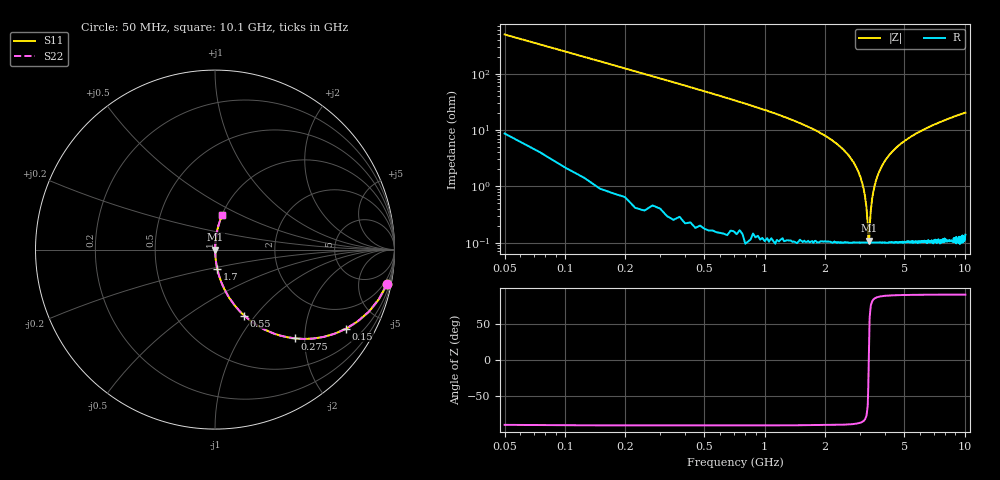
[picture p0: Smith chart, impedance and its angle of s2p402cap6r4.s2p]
! AVX Thin Film Operation		Date: April 2003
! Description: Accu-P® Series, Thin Film, SMD, RF Capacitor
! Part Number: 04025J6R4BBS
! 50 MHz  -  10.05 GHz
! Serial Measurements
# hz S db R 50
!	S11		S21		S12		S22
!	dB	Phase	dB	Phase	dB	Phase	dB	Phase
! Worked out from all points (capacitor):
!   400 points, 50 MHz to 10.1 GHz, reference 50 ohm
!   read as one part in series: C = 6.4 pF near 100 MHz
!   lowest |Z| = 108 mohm at 3.33 GHz (marker M1)
!   series resonance near 3.319 GHz, so ESL is about 360 pH
!   S11 on the Smith chart (normalised r, x): 50 MHz: 1, -10; 150 MHz: 1.02, -3.30; 275 MHz: 1.01, -1.80; 550 MHz: 1.00, -0.88; 1.7 GHz: 1.00, -0.22; 10.1 GHz: 1.00, +0.40
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5e7  -0.20 -11.3  -14.10 77.7  -14.10 77.7  -0.20 -11.3
1.5e8  -1.38 -31.1  -5.75 58.6  -5.75 58.6  -1.38 -31.1
2.75e8  -3.52 -47.9  -2.59 41.8  -2.59 41.8  -3.52 -47.9
5.5e8  -7.92 -66.1  -0.78 23.7  -0.78 23.7  -7.92 -66.1
1.7e9  -19.40 -83.3  -0.06 6.2  -0.06 6.2  -19.40 -83.3
1.73e9  -19.60 -83.4  -0.06 6.0  -0.06 6.0  -19.60 -83.4
2.48e9  -27.00 -86.2  -0.02 2.5  -0.02 2.5  -27.00 -86.2
2.93e9  -34.50 -85.9  -0.01 1.1  -0.01 1.1  -34.50 -85.9
3.18e9  -43.60 -80.9  -0.01 0.4  -0.01 0.4  -43.60 -80.9
3.23e9  -47.40 -76.3  -0.01 0.2  -0.01 0.2  -47.40 -76.3
3.28e9  -53.50 -61.6  -0.01 0.1  -0.01 0.1  -53.50 -61.6
3.3e9  -58.20 -35.5  -0.01 0.0  -0.01 0.0  -58.20 -35.5
3.33e9  -59.30 22.7  -0.01 -0.0  -0.01 -0.0  -59.30 22.7
3.35e9  -54.70 57.0  -0.01 -0.1  -0.01 -0.1  -54.70 57.0
3.4e9  -48.20 74.9  -0.01 -0.2  -0.01 -0.2  -48.20 74.9
3.5e9  -41.80 82.5  -0.01 -0.5  -0.01 -0.5  -41.80 82.5
3.6e9  -38.10 84.7  -0.01 -0.7  -0.01 -0.7  -38.10 84.7
3.9e9  -32.20 86.3  -0.01 -1.4  -0.01 -1.4  -32.20 86.3
5.08e9  -23.70 85.4  -0.03 -3.8  -0.03 -3.8  -23.70 85.4
6.75e9  -18.80 82.9  -0.07 -6.6  -0.07 -6.6  -18.80 82.9
8.43e9  -16.00 80.5  -0.12 -9.1  -0.12 -9.1  -16.00 80.5
1.01e10  -14.10 78.2  -0.18 -11.4  -0.18 -11.4  -14.10 78.2
